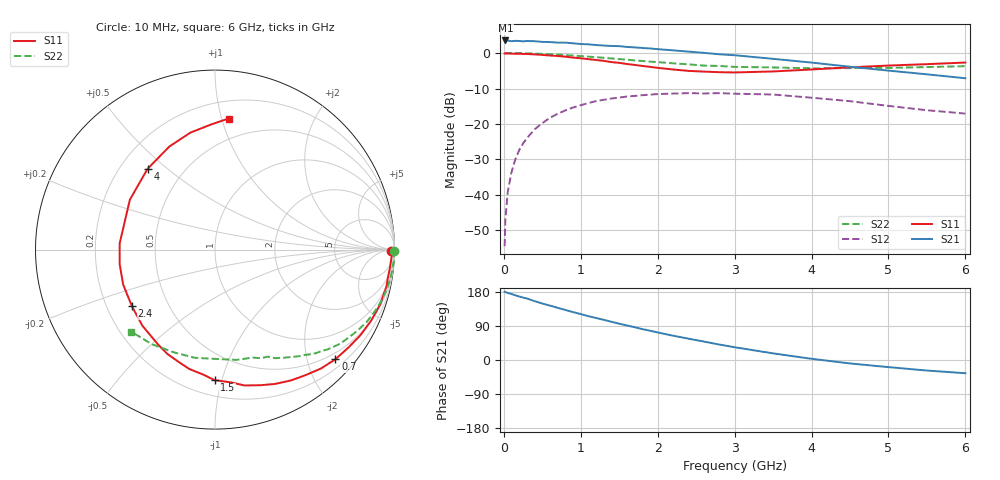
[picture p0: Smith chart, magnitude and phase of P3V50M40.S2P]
! SIEMENS Small Signal Semiconductors
! BFP181
! Si NPN RF Bipolar Junction Transistor in SOT143
! VCE = 0.5 V  IC = 0.4 mA
! Common Emitter S-Parameters:  March  1996
# GHz  S  MA  R  50
!  f  S11  S21  S12  S22
! GHz  MAG  ANG  MAG  ANG  MAG  ANG  MAG  ANG
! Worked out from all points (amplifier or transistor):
!   36 points, 10 MHz to 6 GHz, reference 50 ohm
!   highest |S21| = 3.5 dB at 20 MHz (marker M1)
!   |S21| within 3 dB of that: start of sweep to 2.322 GHz
!   unconditionally stable (mu >= 1): 3.504 GHz to end of sweep
!   at 250 MHz: K = 0.10, MSG = 14.4 dB, |S12| = -25.5 dB
!   at 1.4 GHz: K = 0.52, MSG = 7.4 dB, |S12| = -12.8 dB
!   at 6 GHz: K = 1.73, MAG = 0.0 dB, |S12| = -17.1 dB
!   S11 on the Smith chart (normalised r, x): 10 MHz: 84, -51; 700 MHz: 0.37, -2.54; 1.5 GHz: 0.31, -0.95; 2.4 GHz: 0.31, -0.28; 4 GHz: 0.31, +0.43; 6 GHz: 0.33, +1.05
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0.01  0.9828 -0.6  1.482 179.9  0.0019 84.0  1 -0.3
0.02  0.9877 -1.2  1.503 179.5  0.0045 89.1  0.9959 -0.6
0.05  0.9835 -2.9  1.5 177.1  0.0109 87.7  0.9976 -1.7
0.1  0.9797 -6.2  1.466 174.1  0.0211 85.5  0.9997 -3.3
0.15  0.976 -9.2  1.484 170.8  0.032 83.3  0.9953 -4.9
0.2  0.9772 -12.2  1.477 167.6  0.0429 81.2  0.995 -6.6
0.3  0.9698 -18.3  1.477 162.3  0.0633 76.6  0.9902 -9.8
0.4  0.9563 -24.3  1.468 155.3  0.0839 71.9  0.9814 -13.1
0.7  0.9075 -42.3  1.401 137.7  0.1393 58.8  0.9493 -22.5
0.8  0.8878 -48.2  1.4 132.0  0.1554 54.4  0.9368 -25.4
1.1  0.8199 -65.9  1.326 115.6  0.1974 42.4  0.8888 -33.7
1.5  0.7272 -90.2  1.25 95.8  0.2356 28.1  0.8199 -43.5
1.8  0.6572 -108.1  1.178 81.5  0.2546 19.3  0.7726 -49.4
2.2  0.5862 -133.6  1.091 64.1  0.2683 7.6  0.7161 -57.2
2.4  0.5601 -145.8  1.047 56.3  0.2721 2.1  0.6924 -60.9
2.6  0.5473 -159.3  1.005 48.7  0.269 -2.0  0.6647 -63.8
3  0.5324 176.3  0.931 33.7  0.2674 -11.8  0.6375 -70.7
3.5  0.5498 149.6  0.828 17.5  0.2601 -21.1  0.626 -79.0
4  0.5861 129.9  0.733 3.2  0.2347 -29.7  0.6092 -89.4
4.5  0.6281 113.9  0.641 -9.1  0.2097 -37.2  0.6133 -100.7
5.5  0.6965 92.0  0.501 -27.8  0.1563 -40.9  0.6339 -123.8
6  0.7342 84.1  0.441 -34.9  0.1401 -38.3  0.6528 -135.5
